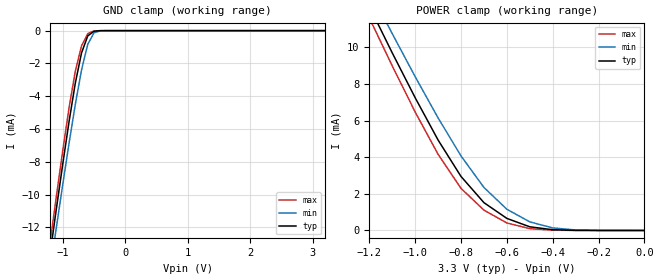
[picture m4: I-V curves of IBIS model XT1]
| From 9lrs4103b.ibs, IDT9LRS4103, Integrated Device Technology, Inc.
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|   Model XT1
[Model]   XT1
Model_type   Input
Polarity   Non-Inverting
Vinl =   0.80V
Vinh =   2.00V
C_comp   3.40pF   2.85pF   3.95pF
[Temperature Range]   27.00   70.00   0.000
[Voltage Range]   3.30V   3.00V   3.70V
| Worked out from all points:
|   GND clamp passes 1 mA (typ) near -0.67 V on its own axis
|   POWER clamp passes 1 mA (typ) near -0.64 V on its own axis
[GND_clamp]
| voltage   I(typ)   I(min)   I(max)
-3.3V     -73.77mA   -71.67mA   -75.17mA
-1.2V     -13.54mA   -14.55mA   -12.85mA
-1.1V     -10.8mA    -11.94mA   -10.04mA
-1V       -8.13mA    -9.38mA    -7.31mA
-900mV    -5.56mA    -6.88mA    -4.72mA
-800mV    -3.21mA    -4.51mA    -2.48mA
-700mV    -1.36mA    -2.4mA     -930uA
-600mV    -320uA     -830uA     -180uA
-500mV    -35.07uA   -130uA     -14.53uA
-400mV    -1.76uA    -10.11uA   -470nA
3.2V      -2.77nA    4.29uA     -450pA
|   3.30   0.000A   0.000A   0.000A
[POWER_clamp]
| voltage   I(typ)   I(min)   I(max)
-3.3V     68.72mA    66.56mA    70.17mA
-1.2V     12.24mA    13.16mA    11.61mA
-1.1V     9.7mA      10.75mA    8.99mA
-1V       7.25mA     8.4mA      6.47mA
-900mV    4.94mA     6.15mA     4.16mA
-800mV    2.95mA     4.07mA     2.3mA
-700mV    1.52mA     2.35mA     1.11mA
-600mV    660uA      1.16mA     410uA
-500mV    200uA      470uA      98.94uA
-400mV    41.76uA    140uA      16.56uA
-300mV    6.4uA      27.64uA    2.03uA
0V        0A         0A         0A
